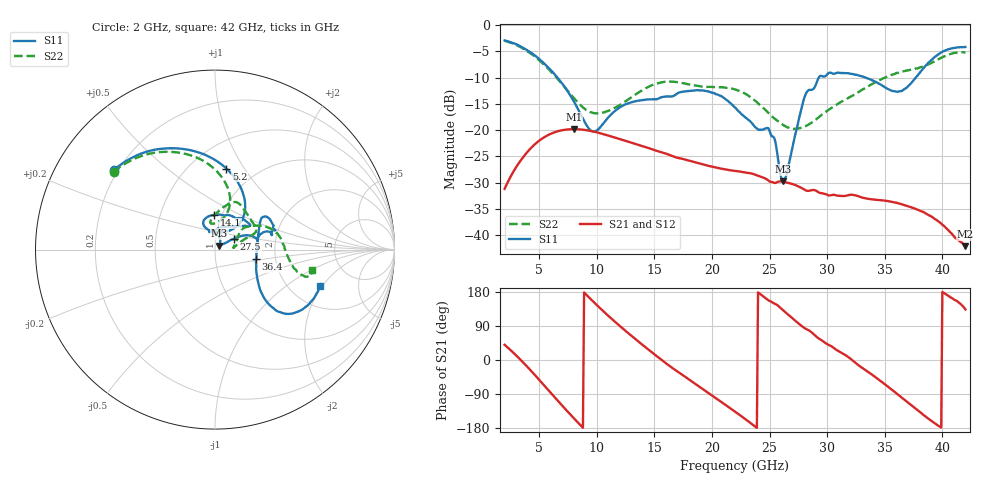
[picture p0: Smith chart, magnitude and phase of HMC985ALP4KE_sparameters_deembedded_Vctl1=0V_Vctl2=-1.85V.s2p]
!s2p File: Measurements: S11, S21, S12, S22
# GHz S dB R 50.0
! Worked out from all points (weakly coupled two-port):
!   401 points, 2 GHz to 42 GHz, reference 50 ohm
!   highest |S21| = -19.81 dB at 8 GHz (marker M1); lowest = -42.1 dB at 42 GHz (marker M2)
!   lowest |S11| = -29.7 dB at 26.2 GHz (marker M3), VSWR 1.07, Z = 52.4 + j2.36 ohm
!   |S11| at or under -10 dB: 6.596 GHz to 29.27 GHz (22.67 GHz wide, 126 % of centre); 33.36 GHz to 37.69 GHz (4.332 GHz wide, 12.2 % of centre)
!   |S22| runs from -19.8 to -2.9 dB; largest |S21 - S12| = 0.00018
!   S11 on the Smith chart (normalised r, x): 2 GHz: 0.18, +0.34; 5.2 GHz: 0.73, +0.84; 14.1 GHz: 0.92, +0.37; 27.5 GHz: 1.22, +0.15; 36.4 GHz: 1.58, -0.18; 42 GHz: 2.90, -1.91
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2  -2.90 141.6  -31.21 40.0  -31.20 40.0  -2.95 142.5
3.6  -4.29 112.3  -25.18 -6.1  -25.18 -6.1  -4.45 114.7
5.2  -6.82 82.0  -21.70 -59.0  -21.70 -59.0  -7.05 89.7
8  -14.47 46.8  -19.81 -153.4  -19.82 -153.4  -13.85 72.6
8.7  -17.41 52.1  -19.89 -175.6  -19.90 -175.6  -15.48 78.7
9.8  -20.29 86.8  -20.31 151.0  -20.32 150.9  -16.78 92.8
12.1  -15.53 113.0  -21.78 87.2  -21.78 87.1  -15.06 95.1
14.1  -14.23 91.1  -23.15 36.7  -23.15 36.7  -12.19 77.7
15.4  -13.94 73.1  -24.07 5.8  -24.08 5.8  -10.98 69.3
19.3  -12.46 34.4  -26.59 -78.7  -26.59 -78.8  -11.67 40.1
22  -15.67 52.3  -27.78 -136.1  -27.79 -136.1  -12.24 22.9
25  -20.10 98.3  -29.79 155.9  -29.79 155.8  -16.94 15.8
26.2  -29.73 43.6  -29.86 130.6  -29.86 130.6  -19.05 8.2
27.5  -18.36 30.0  -30.72 96.6  -30.73 96.6  -19.68 6.7
28.1  -13.33 20.8  -31.45 83.0  -31.45 82.9  -19.28 11.1
28.7  -12.29 12.9  -31.43 71.6  -31.43 71.6  -18.48 17.0
31  -9.06 23.3  -32.52 23.4  -32.53 23.3  -14.88 36.5
33.3  -9.95 34.3  -33.00 -25.9  -33.03 -26.0  -11.99 31.7
35.4  -12.27 12.2  -33.59 -73.3  -33.60 -73.3  -9.65 20.9
36.4  -12.58 -13.0  -34.09 -97.4  -34.10 -97.5  -8.88 14.3
39.5  -5.80 -43.3  -37.13 -170.2  -37.16 -170.5  -6.64 -14.0
42  -4.14 -19.0  -42.14 133.4  -42.15 133.2  -5.16 -11.6
